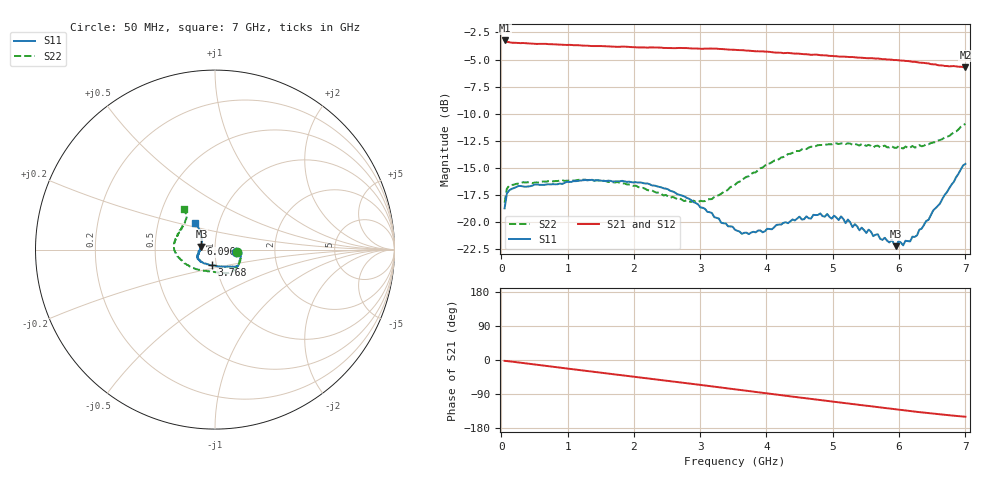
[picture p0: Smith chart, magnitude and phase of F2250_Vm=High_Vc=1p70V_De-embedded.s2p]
! Integrated Device Technology
! Corporate Headquarters
! 6024 Silver Creek Valley Road
! San Jose, CA 95138  USA
! Phone:  1-408-284-8200
! Toll Free:  1-800-223-1366
! Webpage:  http://www.idt.com/
! Timing and RF Division
! 515 Groton Road, Suite 102
! Westford, MA 01886-6024
! Device:  F2250
! Description: Voltage Variable RF Attenuator
! Frequency:  50.0 -  6000.00 MHz
! Package:  3x3 mm Thin QFN Plastic Package: 16 pin
! Ports:  2 RF, 3 DC
!  Pin  1  = GND
!  Pin  2  = NC
!  Pin  3  = RF1  = Port 1
!  Pin  4  = NC
!  Pin  5  = GND
!  Pin  6  = GND
!  Pin  7  = GND
!  Pin  8  = GND
!  Pin  9  = NC
!  Pin 10  = RF2  = Port 2
!  Pin 11  = NC
!  Pin 12  = GND
!  Pin 13  = GND
!  Pin 14  = VCNTRL
!  Pin 15  = VDD
!  Pin 16  = VMODE
! Vcntrl:  1.700 Volts
! Vmode:  +3.300 Volts
! Vdd:  +3.30  Volts
! Current:  1.326 mA
! Data:  The device was measured on a the F2250 evaluation board which has
!  individual transmission lines to the RF pins.  Data was collected
!  using a calibrated network analyzer.  The evaluation board was
!  de-embedded using a TRL calibration technique.
!  The reference plane is the edge of the package pin.
! Misc:  SN 10
!  Action Tracker AT0258
! Date Measured:  2014-11-26
! Date:  2015-10-15  MJV
! Note:
!  Integrated Device Technology supplies this data as a sample of measured
!  data at the package pin for this product.  Your particular data for this
!  product may vary.
!  Data was taken at 25 degrees C.
!  Integrated Device Technology reserves the right to change this data at anytime.
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# GHz S dB R 50
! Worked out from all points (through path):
!   201 points, 50 MHz to 7 GHz, reference 50 ohm
!   highest |S21| = -3.24 dB at 50 MHz (marker M1); lowest = -5.7 dB at 7 GHz (marker M2)
!   group delay of S21, straight-line fit = 60.1 ps
!   lowest |S11| = -22.2 dB at 5.957 GHz (marker M3), VSWR 1.17, Z = 42.9 + j1.47 ohm
!   |S11| at or under -10 dB: start of sweep to end of sweep
!   |S22| runs from -18.2 to -10.9 dB; largest |S21 - S12| = 0.0036
!   S11 on the Smith chart (normalised r, x): 50 MHz: 1.26, -0.03; 3.768 GHz: 0.95, -0.17; 6.096 GHz: 0.86, +0.05; 7 GHz: 0.77, +0.24
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0.05  -18.72 -5.7  -3.24 -2.3  -3.24 -2.3  -18.20 -6.7
0.08475  -17.33 -4.4  -3.36 -2.7  -3.37 -2.7  -16.89 -5.4
0.2585  -16.65 -8.6  -3.48 -6.4  -3.48 -6.4  -16.43 -11.8
1.2315  -16.12 -31.8  -3.72 -27.7  -3.70 -27.7  -16.07 -45.6
2.37825  -16.73 -40.8  -3.90 -52.0  -3.90 -52.0  -17.26 -71.9
2.969  -18.36 -51.2  -3.99 -65.0  -4.00 -65.0  -18.13 -98.8
3.525  -20.69 -82.5  -4.11 -77.4  -4.12 -77.5  -16.54 -132.6
3.76825  -20.94 -102.4  -4.20 -82.9  -4.20 -82.9  -15.55 -145.0
4.4285  -19.83 -138.7  -4.45 -97.4  -4.44 -97.5  -13.43 -169.9
4.7065  -19.31 -149.4  -4.56 -103.5  -4.56 -103.5  -13.06 -176.8
5.1235  -19.45 -159.8  -4.74 -112.5  -4.71 -112.5  -12.73 172.9
5.29725  -20.44 -163.9  -4.77 -116.1  -4.78 -116.2  -12.85 169.3
5.5405  -20.67 -173.5  -4.88 -121.4  -4.87 -121.5  -12.86 162.6
5.85325  -21.85 174.3  -5.00 -128.0  -5.02 -128.1  -13.09 154.3
5.888  -21.61 173.9  -5.01 -128.8  -5.04 -128.8  -12.98 154.5
5.9575  -22.20 167.3  -5.05 -130.2  -5.04 -130.3  -13.14 151.6
5.99225  -21.71 165.5  -5.07 -131.1  -5.07 -131.2  -12.99 151.2
6.06175  -22.12 161.1  -5.10 -132.4  -5.11 -132.5  -13.20 148.4
6.0965  -21.70 158.4  -5.13 -133.3  -5.12 -133.3  -13.02 147.8
6.27025  -21.20 146.5  -5.24 -136.8  -5.24 -136.9  -13.07 141.7
6.75675  -16.86 128.4  -5.63 -145.8  -5.62 -145.9  -12.04 129.4
7  -14.62 126.7  -5.73 -149.7  -5.75 -149.8  -10.93 127.3
